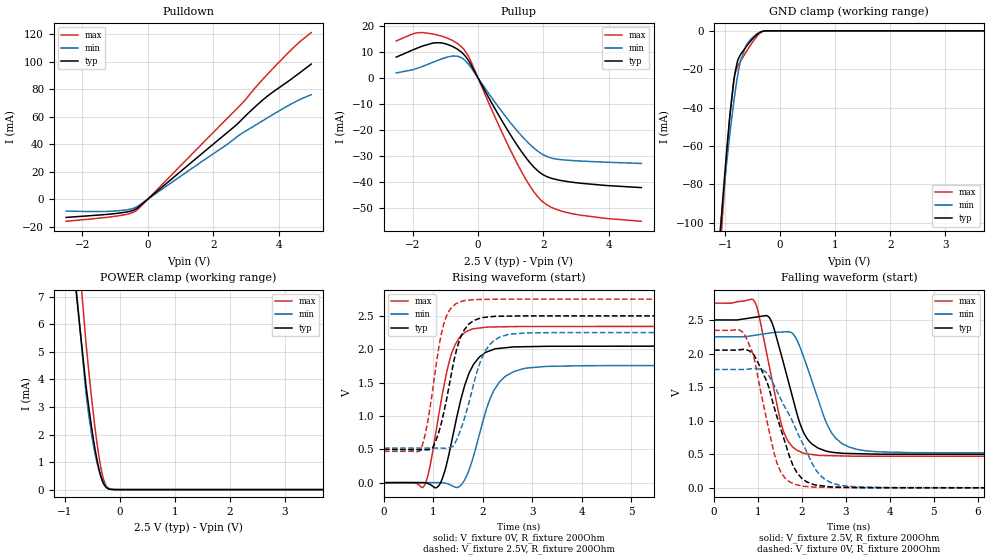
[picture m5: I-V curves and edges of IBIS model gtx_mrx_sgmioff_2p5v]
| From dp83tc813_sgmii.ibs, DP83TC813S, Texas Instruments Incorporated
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| gtx_mrx_sgmii_off_2p5v
[Model]   gtx_mrx_sgmioff_2p5v
Model_type   I/O
Polarity   Non-Inverting
Enable   Active-Low
Vinl = 0.7
Vinh = 1.7
Vmeas = 1.25
Vref = 1.25
Cref = 2pF
Rref = 100000
|   typ   min   max
C_comp   4.12pF   3.94pF   4.21pF
[Voltage Range]   2.5   2.25   2.75
[Temperature Range]   27   150   -40
[Pullup Reference]   2.5   2.25   2.75
[Pulldown Reference]   -0   -0   0
[Power Clamp Reference]   2.5   2.25   2.75
[GND Clamp Reference]   0   0   0
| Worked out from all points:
|   slope of the pulldown table from 0 to 0.375 V, typ, clamps not added: 49.7 ohm
|   slope of the pullup table from 0 to 0.375 V, typ, clamps not added: 43.5 ohm
|   GND clamp passes 1 mA (typ) near -0.38 V on its own axis
|   POWER clamp passes 1 mA (typ) near -0.41 V on its own axis
|   falling waveform, V_fixture 2.5V, R_fixture 200Ohm: 20-80 % time 510ps typ, 572ps min, 434ps max; typ from 2.5 V to 0.498 V
|   rising waveform, V_fixture 0V, R_fixture 200Ohm: 20-80 % time 411ps typ, 454ps min, 356ps max; typ from 0 V to 2.05 V
|   rising waveform, V_fixture 2.5V, R_fixture 200Ohm: 20-80 % time 351ps typ, 418ps min, 294ps max; typ from 0.498 V to 2.5 V
|   falling waveform, V_fixture 0V, R_fixture 200Ohm: 20-80 % time 590ps typ, 788ps min, 458ps max; typ from 2.05 V to 0 V
[Pulldown]
|   Voltage   I(typ)   I(min)   I(max)
-2.5V     -13.29mA   -8.687mA   -16.1mA
-925mV    -10.31mA   -8.492mA   -12.22mA
-512.5mV  -8.603mA   -7.139mA   -10.18mA
-347.5mV  -6.835mA   -5.631mA   -8.211mA
2.638V    52.57mA    43.69mA    63.75mA
2.885V    58.13mA    47.96mA    69.7mA
3.462V    71.02mA    56.29mA    85.76mA
3.958V    80.11mA    63.42mA    98.27mA
4.633V    91.66mA    72.28mA    114.2mA
5V        98.27mA    76.01mA    121.2mA
[GND Clamp]
|   Voltage   I(typ)   I(min)   I(max)
-2.5V     -712.2mA   -617mA     -795.7mA
-1.105V   -112.1mA   -109mA     -122.5mA
-1.045V   -89.14mA   -90.27mA   -96.16mA
-970mV    -62.33mA   -68.65mA   -65.01mA
-910mV    -43.44mA   -53.04mA   -43.24mA
-842.5mV  -26.37mA   -37.26mA   -25.92mA
-782.5mV  -16.71mA   -25.15mA   -19.21mA
-722.5mV  -12.49mA   -15.9mA    -16.01mA
-617.5mV  -8.274mA   -7.642mA   -11.03mA
-497.5mV  -4.092mA   -3.395mA   -5.748mA
-355mV    -617.9uA   -659.9uA   -973.5uA
5V        0A         0A         0A
[Pullup]
|   Voltage   I(typ)   I(min)   I(max)
-2.5V     7.944mA    1.866mA    14.16mA
-1.847V   11.46mA    3.685mA    17.29mA
-1.315V   13.45mA    6.279mA    16.67mA
-752.5mV  11.89mA    8.383mA    14.16mA
-460mV    9.358mA    7.341mA    11.34mA
-257.5mV  5.988mA    4.704mA    7.488mA
642.5mV   -14.55mA   -11.48mA   -18.41mA
1.272V    -27.27mA   -21.43mA   -34.67mA
1.677V    -33.87mA   -26.64mA   -43.23mA
2.007V    -37.38mA   -29.68mA   -47.93mA
2.953V    -40.27mA   -31.88mA   -52.42mA
5V        -42.22mA   -32.93mA   -55.18mA
[POWER Clamp]
|   Voltage   I(typ)   I(min)   I(max)
-2.5V     111.4mA    76.19mA    154.9mA
-1.06V    12.26mA    13.09mA    16.05mA
-617.5mV  3.803mA    3.522mA    5.367mA
-557.5mV  2.879mA    2.591mA    4.147mA
-505mV    2.141mA    1.896mA    3.157mA
-445mV    1.398mA    1.242mA    2.137mA
-392.5mV  857.5uA    791.9uA    1.369mA
-347.5mV  495.5uA    495.6uA    828.3uA
-302.5mV  241.6uA    280.6uA    419.5uA
-220mV    36.62uA    73.16uA    55.78uA
-2.5mV    0A         192.6nA    0A
5V        0A         0A         0A
[Ramp]
R_load = 200
|   typ   min   max
dV/dt_r   1.23008/4.10787e-10   1.05676/4.50234e-10   1.40675/3.56008e-10
dV/dt_f   1.20124/5.07103e-10   1.03898/5.70688e-10   1.36857/4.32598e-10
[Falling Waveform]
V_fixture = 2.5V
V_fixture_min = 2.25V
V_fixture_max = 2.75V
R_fixture = 200Ohm
C_fixture = 0F
|   Time   V(typ)   V(min)   V(max)
0s        2.5V       2.25V      2.75V
889.7ps   2.536V     2.268V     2.801V
1.018ns   2.549V     2.281V     2.577V
1.257ns   2.534V     2.304V     1.805V
1.587ns   1.838V     2.322V     828.7mV
1.806ns   1.298V     2.285V     598.2mV
2.021ns   845.9mV    1.979V     519.6mV
2.645ns   534.6mV    850.1mV    479.3mV
3.252ns   508.8mV    572.5mV    471.5mV
12ns      497.9mV    518.3mV    469mV
[Rising Waveform]
V_fixture = 0V
V_fixture_min = 0V
V_fixture_max = 0V
R_fixture = 200Ohm
C_fixture = 0F
|   Time   V(typ)   V(min)   V(max)
0s        12.18uV    94.32uV    6.791uV
816.9ps   352.5uV    284.5uV    -45.21mV
929.9ps   -26.62mV   310.8uV    239.2mV
1.113ns   -42.15mV   353.4uV    1.038V
1.372ns   626mV      -45.2mV    1.943V
1.563ns   1.268V     -34.9mV    2.202V
1.789ns   1.739V     341.1mV    2.303V
2.228ns   1.999V     1.387V     2.333V
2.851ns   2.037V     1.712V     2.34V
12ns      2.05V      1.761V     2.345V
[Rising Waveform]
V_fixture = 2.5V
V_fixture_min = 2.25V
V_fixture_max = 2.75V
R_fixture = 200Ohm
C_fixture = 0F
|   Time   V(typ)   V(min)   V(max)
0s        497.9mV    518.3mV    469mV
740.7ps   493.2mV    518.7mV    492.1mV
984.9ps   523.2mV    518.8mV    1.39V
1.12ns    782.2mV    518.8mV    2.07V
1.241ns   1.158V     513.7mV    2.45V
1.401ns   1.773V     548.1mV    2.647V
1.587ns   2.235V     870.1mV    2.722V
2.027ns   2.476V     1.945V     2.746V
2.533ns   2.496V     2.222V     2.749V
12ns      2.5V       2.25V      2.75V
[Falling Waveform]
|Gnd
V_fixture = 0V
V_fixture_min = 0V
V_fixture_max = 0V
R_fixture = 200Ohm
C_fixture = 0F
|   Time   V(typ)   V(min)   V(max)
0s        2.051V     1.763V     2.345V
634.7ps   2.06V      1.762V     2.328V
904.6ps   1.98V      1.775V     1.943V
1.18ns    1.612V     1.723V     1.066V
1.43ns    1.06V      1.441V     370.9mV
1.605ns   696.1mV    1.21V      153.2mV
1.867ns   247.4mV    866.6mV    46.61mV
2.402ns   35.08mV    194.6mV    9.991mV
2.892ns   10.14mV    36.2mV     2.993mV
12ns      12.27uV    94.53uV    6.91uV
